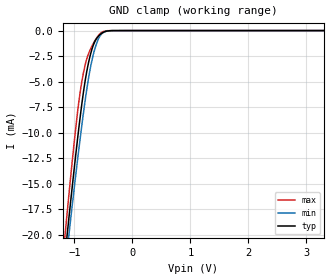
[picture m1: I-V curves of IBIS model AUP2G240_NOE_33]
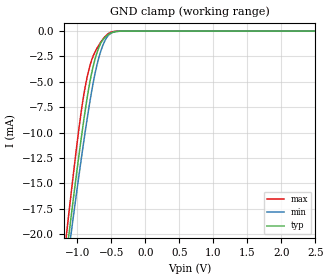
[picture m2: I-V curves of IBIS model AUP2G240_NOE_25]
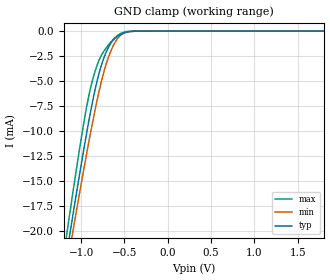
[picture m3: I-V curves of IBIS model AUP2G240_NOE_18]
| TEXAS INSTRUMENTS INCORPORATED
| Standard Linear and Logic Group
| IBIS Model of SN74AUP2G240
| LOW-POWER DUAL BUFFER/DRIVER WITH 3-STATE OUTPUTS
| This file contains package information for the following:
|  WCSP 8-pin (YFP_YZP) package as [Component] AUP2G240_YFP_YZP
|  SSOP 8-pin (DCU) package as [Component] AUP2G240_DCU
| This device can be powered at the following Vccs:
|  3.3 volt Vcc
|  2.5 volt Vcc
|  1.8 volt Vcc
|  1.5 volt Vcc
|  1.2 volt Vcc
|  0.8 volt Vcc
| This file provides unique models under the [Model Selector] for each Vcc.
| For operation at a specific Vcc, select the appropriate model after each
| [Model Selector] keyword.
[IBIS Ver]   3.2
[Comment char]  |_char
[File Name]   sn74aup2g240.ibs
[File Rev]   1.0 | b_die
[Date]   June 10, 2010
[Source]   Data created from TI-SPICE simulations at TI-SLL.
[Notes]   The following is an IBIS list for the SN74AUP2G240.
   Please contact sllibis@ti.com with questions and
   comments concerning SLL IBIS models.
   -FILE REV HISTORY
   -1.0 Release IBIS file on 06/16/10.
   -Power Clamp data deleted from control input model as there
   is no power-clamp diode.
[Disclaimer] Property of Texas Instruments Incorporated.  Unauthorized
   reproduction and/or distribution is strictly prohibited.
   This product is protected under copyright law.
   Created  2010, (C) Copyright  2010, Texas Instruments
   UNLESS THERE IS A SIGNED, WRITTEN AGREEMENT TO THE
   CONTRARY, TEXAS INSTRUMENTS (TI) IS PROVIDING THE IBIS
   MODELS  AND WITHOUT ANY WARRANTY, EXPRESSED OR
   IMPLIED.  TI assumes no liability for:
   1) the accuracy of the IBIS models provided to your
   company;
   2) the proper functioning of these IBIS Models in your
   design or for any resulting applications; or
   3) infringement of patents, copyrights or intellectual
   property rights resulting from your use of these IBIS
   models.
   TI provides IBIS Models as a service to our customers.
   You and your company shall not distribute, sell or give
   these models to anyone else without prior written
   permission from TI.
   TI reserves the right to make changes to our products or
   to discontinue any semiconductor product or service
   without notice, and advises our customers to obtain the
   latest version of relevant information to verify, before
   placing orders, that the information being relied on is
   current.
   Please be aware that your receipt and use of the IBIS
   information provided shall serve as acceptance of these
   terms and conditions.  If you do not accept these terms,
   you should return or destroy the IBIS models and any
   other accompanying information immediately.
[Copyright]
| (C) Copyright 2000 Texas Instruments Incorporated. All rights reserved.
| All other rights are reserved.
| Component SN74AUP2G240_YFP_YZP 8-PIN WCSP
[Component]   SN74AUP2G240_YFP_YZP
[Manufacturer]   Texas Instruments, Inc.
[Package]
|   typ   min   max
R_pkg   1.000e-03   1.000e-03   4.000e-03
L_pkg   6.400e-11   2.400e-11   3.790e-10
C_pkg   5.800e-14   0.000e+00   6.700e-14
[Pin]   signal_name   model_name   R_pin   L_pin   C_pin
1   1NOE   AUP2G240_NOE   1.000e-03   2.500e-11   6.400e-14
2   1A   AUP2G240_A   1.000e-03   2.400e-11   6.700e-14
3   2Y   AUP2G240_Y   1.000e-03   2.400e-11   6.700e-14
4   GND   GND   1.000e-03   2.500e-11   6.400e-14
5   2A   AUP2G240_A   1.000e-03   2.500e-11   6.400e-14
6   1Y   AUP2G240_Y   1.000e-03   2.400e-11   6.700e-14
7   2NOE   AUP2G240_NOE   1.000e-03   2.400e-11   6.700e-14
8   VCC   POWER   1.000e-03   2.500e-11   6.400e-14
| Component SN74AUP2G240_DCU 8-PIN SSOP
[Component]   SN74AUP2G240_DCU
[Manufacturer]   Texas Instruments, Inc.
[Package]
|   typ   min   max
R_pkg   2.600e-02   2.300e-02   3.800e-02
L_pkg   1.394e-09   1.066e-09   2.046e-09
C_pkg   2.590e-13   2.150e-13   3.720e-13
[Pin]   signal_name   model_name   R_pin   L_pin   C_pin
1   1NOE   AUP2G240_NOE   2.400e-02   1.520e-09   2.710e-13
2   1A   AUP2G240_A   2.300e-02   1.112e-09   2.180e-13
3   2Y   AUP2G240_Y   2.300e-02   1.070e-09   2.170e-13
4   GND   GND   2.700e-02   2.046e-09   3.720e-13
5   2A   AUP2G240_A   2.700e-02   1.542e-09   2.730e-13
6   1Y   AUP2G240_Y   2.300e-02   1.100e-09   2.240e-13
7   2NOE   AUP2G240_NOE   2.300e-02   1.066e-09   2.150e-13
8   VCC   POWER   3.800e-02   1.696e-09   2.800e-13
| Model AUP2G240_NOE
[Model Selector]   AUP2G240_NOE
AUP2G240_NOE_33   3.3 volt Vcc
AUP2G240_NOE_25   2.5 volt Vcc
AUP2G240_NOE_18   1.8 volt Vcc
AUP2G240_NOE_15A   1.5 volt Vcc
AUP2G240_NOE_12   1.2 volt Vcc
AUP2G240_NOE_08   0.8 volt Vcc
| Model AUP2G240_A
[Model Selector]   AUP2G240_A
AUP2G240_A_33   3.3 volt Vcc
AUP2G240_A_25   2.5 volt Vcc
AUP2G240_A_18   1.8 volt Vcc
AUP2G240_A_15A   1.5 volt Vcc
AUP2G240_A_12   1.2 volt Vcc
AUP2G240_A_08   0.8 volt Vcc
| Model AUP2G240_Y
[Model Selector]   AUP2G240_Y
AUP2G240_Y_33   3.3 volt Vcc
AUP2G240_Y_25   2.5 volt Vcc
AUP2G240_Y_18   1.8 volt Vcc
AUP2G240_Y_15A   1.5 volt Vcc
AUP2G240_Y_12   1.2 volt Vcc
AUP2G240_Y_08   0.8 volt Vcc
| Models and submodels in the file (18): AUP2G240_NOE_33 (Input), AUP2G240_NOE_25 (Input), AUP2G240_NOE_18 (Input), AUP2G240_NOE_15A (Input), AUP2G240_NOE_12 (Input), AUP2G240_NOE_08 (Input), AUP2G240_A_33 (Input), AUP2G240_A_25 (Input), AUP2G240_A_18 (Input), AUP2G240_A_15A (Input), AUP2G240_A_12 (Input), AUP2G240_A_08 (Input), AUP2G240_Y_33 (3-state), AUP2G240_Y_25 (3-state), AUP2G240_Y_18 (3-state), AUP2G240_Y_15A (3-state), AUP2G240_Y_12 (3-state), AUP2G240_Y_08 (3-state)
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[Model]   AUP2G240_NOE_33
Model_type  Input
Vinl=0.9
Vinh=2.1
| variable   typ   min   max
C_comp   1.36pF   1.14pF   1.80pF
[Temperature Range]   40   100   -40
| Ambient temperature   25   85   -40
[Voltage range]   3.3   3   3.6
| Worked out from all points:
|   GND clamp passes 1 mA (typ) near -0.64 V on its own axis
[GND Clamp]
| AUP2G240_NOE_33
|   Voltage   I(typ)   I(min)   I(max)
-3.6V     -169.6mA   -161.4mA   -179.1mA
-1.16V    -21.94mA   -23.37mA   -19.97mA
-1.11V    -19.21mA   -20.81mA   -17.01mA
-1.085V   -17.86mA   -19.54mA   -15.55mA
-940mV    -10.37mA   -12.43mA   -7.747mA
-890mV    -8.015mA   -10.11mA   -5.65mA
-835mV    -5.697mA   -7.708mA   -3.904mA
-755mV    -3.121mA   -4.644mA   -2.253mA
-675mV    -1.456mA   -2.384mA   -1.277mA
-595mV    -617.3uA   -936.6uA   -546.7uA
-515mV    -215.4uA   -247.8uA   -134.4uA
3.3V      132.2pA    540pA      36.28pA
[Model]   AUP2G240_NOE_25
Model_type  Input
Vinl=0.7
Vinh=1.6
| variable   typ   min   max
C_comp   1.40pF   1.19pF   1.79pF
[Temperature Range]   40   100   -40
| Ambient temperature   25   85   -40
[Voltage range]   2.5   2.3   2.7
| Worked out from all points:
|   GND clamp passes 1 mA (typ) near -0.64 V on its own axis
[GND Clamp]
| AUP2G240_NOE_25
|   Voltage   I(typ)   I(min)   I(max)
-3.6V     -169.6mA   -161.4mA   -179.1mA
-1.175V   -22.77mA   -24.14mA   -20.86mA
-1.15V    -21.39mA   -22.85mA   -19.37mA
-1.125V   -20.02mA   -21.57mA   -17.89mA
-1.105V   -18.94mA   -20.55mA   -16.71mA
-1.08V    -17.59mA   -19.29mA   -15.26mA
-950mV    -10.86mA   -12.9mA    -8.222mA
-840mV    -5.891mA   -7.919mA   -4.043mA
-765mV    -3.388mA   -4.989mA   -2.404mA
-680mV    -1.535mA   -2.5mA     -1.33mA
-525mV    -251.7uA   -297.2uA   -166.6uA
2.5V      104.3pA    491.5pA    26.71pA
[Model]   AUP2G240_NOE_18
Model_type  Input
Vinl=0.6825
Vinh=1.0725
| variable   typ   min   max
C_comp   1.44pF   1.25pF   1.79pF
[Temperature Range]   40   100   -40
| Ambient temperature   25   85   -40
[Voltage range]   1.8   1.65   1.95
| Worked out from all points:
|   GND clamp passes 1 mA (typ) near -0.64 V on its own axis
[GND Clamp]
| AUP2G240_NOE_18
|   Voltage   I(typ)   I(min)   I(max)
-3.6V     -169.6mA   -161.4mA   -179.1mA
-1.16V    -21.94mA   -23.37mA   -19.97mA
-1.135V   -20.57mA   -22.08mA   -18.48mA
-1.11V    -19.21mA   -20.81mA   -17.01mA
-1.09V    -18.13mA   -19.79mA   -15.84mA
-960mV    -11.36mA   -13.37mA   -8.712mA
-850mV    -6.292mA   -8.346mA   -4.331mA
-780mV    -3.816mA   -5.529mA   -2.655mA
-700mV    -1.885mA   -2.995mA   -1.553mA
-615mV    -767.6uA   -1.228mA   -703.5uA
-540mV    -313.1uA   -387.9uA   -224.9uA
1.8V      83.14pA    450.9pA    18.98pA
